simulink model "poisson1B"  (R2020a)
settings: Solver=FixedStepDiscrete  StartTime=0.0  StopTime=100  FixedStep=0.01  MaxStep=0.01  RelTol=1e-3  EnableMultiTasking=on

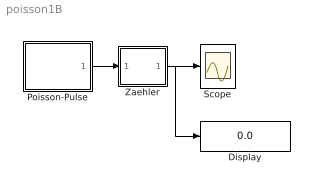
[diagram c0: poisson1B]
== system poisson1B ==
  Display : Display
  Poisson-Pulse : Subsystem  mask{lambda=0.8}
  Scope : Scope
  Zaehler : Subsystem  mask(Vorwaertszaehler){z0=0}
      mask prompts: z0 "Anfangswert"
      mask help: Einfacher Vorwaertszaehler, getriggert durch Signalabfall
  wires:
  Zaehler/1(Out) -> Display/1, Scope/1
  Poisson-Pulse/1(Out) -> Zaehler/1(In)

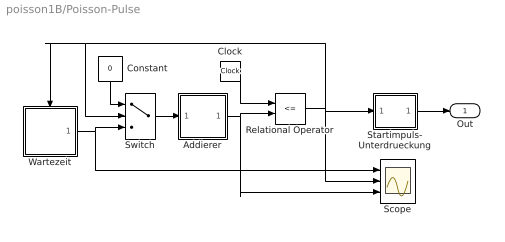
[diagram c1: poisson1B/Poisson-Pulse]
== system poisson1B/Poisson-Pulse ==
  Addierer : Subsystem
  Clock : Clock
  Constant : Constant  Value=0
  Relational Operator : RelationalOperator  Operator=<=  OutDataTypeStr=boolean
  Scope : Scope  NumInputPorts=3
  Startimpuls- Unterdrueckung : Subsystem
  Switch : Switch  Threshold=1
  Wartezeit : Subsystem
  Out : Outport
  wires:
  Clock/1 -> Relational Operator/1
  Relational Operator/1 -> Scope/2, Wartezeit/Trigger, Switch/2, Startimpuls- Unterdrueckung/1(In)
  Wartezeit/1(dt) -> Scope/1, Switch/3
  Addierer/1(Summe) -> Relational Operator/2, Scope/3
  Startimpuls- Unterdrueckung/1(Out) -> Out/1
  Switch/1 -> Addierer/1(In)
  Constant/1 -> Switch/1

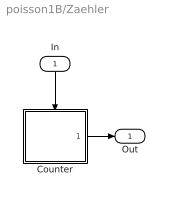
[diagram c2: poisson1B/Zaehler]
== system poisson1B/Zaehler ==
  In : Inport
  Counter : Subsystem
  Out : Outport
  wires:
  Counter/1(Out) -> Out/1
  In/1 -> Counter/Trigger

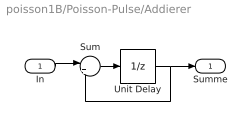
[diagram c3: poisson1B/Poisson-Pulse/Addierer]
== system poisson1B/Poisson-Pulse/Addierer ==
  In : Inport
  Sum : Sum  Inputs=|++
  Unit Delay : UnitDelay  SampleTime=-1  HasFrameUpgradeWarning=on
  Summe : Outport
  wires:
  In/1 -> Sum/1
  Unit Delay/1 -> Sum/2, Summe/1
  Sum/1 -> Unit Delay/1

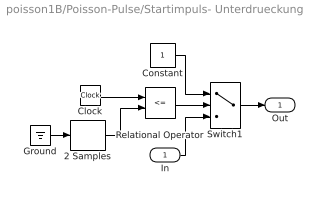
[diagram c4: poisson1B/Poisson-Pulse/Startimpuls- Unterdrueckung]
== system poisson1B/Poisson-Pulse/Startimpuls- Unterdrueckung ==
  In : Inport
  2 Samples : SampleTimeMath  TsampMathOp=Ts Only  weightValue=2
  Clock : Clock
  Constant : Constant
  Ground : Ground
  Relational Operator : RelationalOperator  Operator=<=  OutDataTypeStr=boolean
  Switch1 : Switch  Threshold=1
  Out : Outport
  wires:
  Ground/1 -> 2 Samples/1
  2 Samples/1 -> Relational Operator/2
  Clock/1 -> Relational Operator/1
  Switch1/1 -> Out/1
  Relational Operator/1 -> Switch1/2
  Constant/1 -> Switch1/1
  In/1 -> Switch1/3

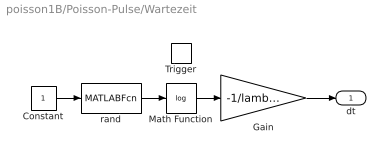
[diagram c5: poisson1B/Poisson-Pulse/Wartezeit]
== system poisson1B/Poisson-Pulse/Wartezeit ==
  Trigger : TriggerPort  TriggerType=falling  VariantControl=Variant
  Constant : Constant
  Gain : Gain  Gain=-1/lambda
  Math Function : Math  Operator=log  SignedPower=on
  rand : MATLABFcn  MATLABFcn=rand
  dt : Outport
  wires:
  rand/1 -> Math Function/1
  Math Function/1 -> Gain/1
  Gain/1 -> dt/1
  Constant/1 -> rand/1

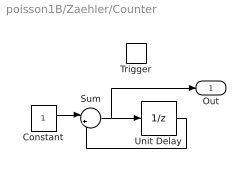
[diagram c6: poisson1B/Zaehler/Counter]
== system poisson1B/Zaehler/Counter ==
  Trigger : TriggerPort  TriggerType=falling  VariantControl=Variant
  Constant : Constant
  Sum : Sum  Inputs=|++
  Unit Delay : UnitDelay  InitialCondition=z0  SampleTime=-1  HasFrameUpgradeWarning=on
  Out : Outport  InitialOutput=z0
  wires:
  Constant/1 -> Sum/1
  Sum/1 -> Unit Delay/1, Out/1
  Unit Delay/1 -> Sum/2
